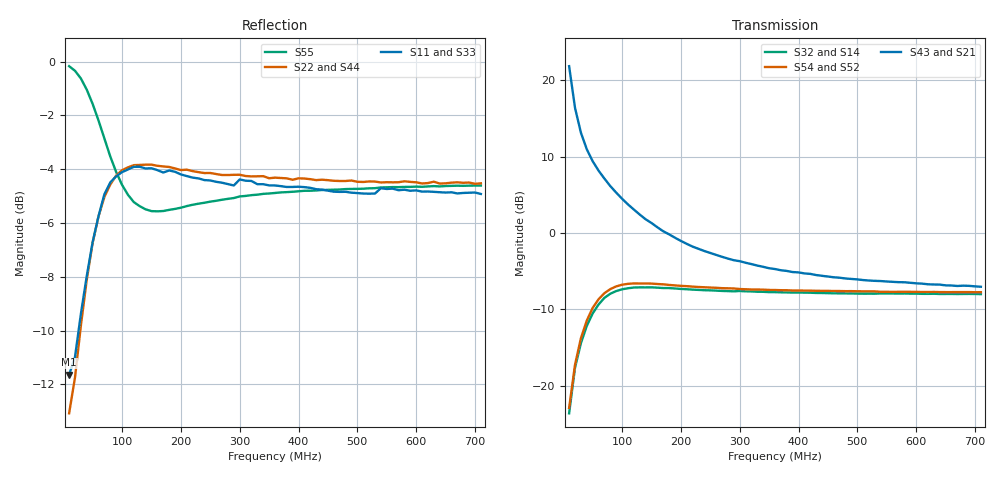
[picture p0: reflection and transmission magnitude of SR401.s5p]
!  POLYFET RF DEVICES
!  S PARAMETERS FOR
!  SR401 (EACH SIDE)
!  VDS=28, IDQ=600MA
! Date: Mon Jan 21 15:37:56 2002
!AWR Design Environment (2053) Wed Feb 04 15:55:06 2004
!freq-unit  param-type  data-format  keyword  impedance-ohms
# MHz  S  MA  R  50
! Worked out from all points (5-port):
!   71 points, 10 MHz to 710 MHz, reference 50 ohm
!   strongest paths, dB at 10 MHz, 180 MHz, 360 MHz, 540 MHz, 710 MHz:
!     S43: 21.9, -0.2, -4.7, -6.3, -7.0
!     S21: 21.9, -0.2, -4.7, -6.3, -7.0
!     S54: -22.9, -6.8, -7.5, -7.7, -7.7
!     S52: -22.9, -6.8, -7.5, -7.7, -7.7
!     S32: -23.6, -7.2, -7.7, -7.9, -8.0
!     S14: -23.6, -7.2, -7.7, -7.9, -8.0
!   lowest |S11| = -11.6 dB at 10 MHz (marker M1), VSWR 1.71, Z = 50.4 - j27.2 ohm
!   |S11| at or under -10 dB: start of sweep to 26.11 MHz
